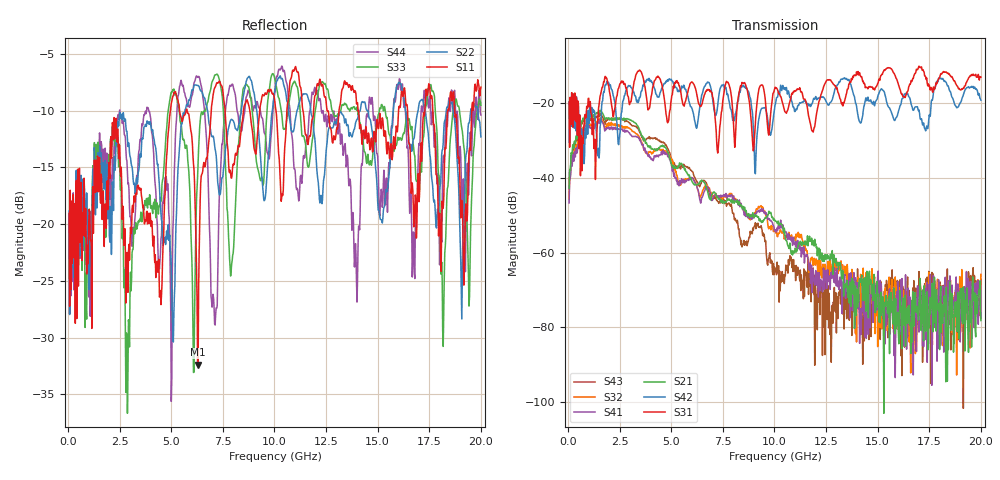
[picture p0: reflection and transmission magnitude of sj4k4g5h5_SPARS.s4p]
! FILE: E:\users\goganessyan\GBX_Backplane\FR408_backplane\1m_INBOUND_FEXT\sj4k4g5h5_SPARS.s4p
# MHZ S RI R 50.00
! FREQ  S11  S12  S13  S14
!  S21  S22  S23  S24
!  S31  S32  S33  S34
!  S41  S42  S43  S44
!  REAL  IMAG  REAL  IMAG  REAL  IMAG  REAL  IMAG
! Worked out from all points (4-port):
!   799 points, 50 MHz to 20 GHz, reference 50 ohm
!   strongest paths, dB at 50 MHz, 5.025 GHz, 10.03 GHz, 15.03 GHz, 20 GHz:
!     S31: -19.7, -18.0, -15.8, -14.5, -13.1
!     S42: -19.7, -14.0, -20.7, -17.8, -19.2
!     S21: -42.8, -36.8, -51.5, -71.4, -78.2
!     S41: -46.7, -37.2, -54.1, -65.0, -77.5
!     S32: -45.6, -35.0, -53.9, -71.4, -65.8
!     S43: -42.8, -35.3, -64.3, -68.4, -67.1
!   lowest |S11| = -32.4 dB at 6.275 GHz (marker M1), VSWR 1.05, Z = 51.9 - j1.58 ohm
!   |S11| at or under -10 dB: start of sweep to 4.959 GHz; 5.768 GHz to 6.936 GHz (1.168 GHz wide, 18.4 % of centre); 14.05 GHz to 16.01 GHz (1.965 GHz wide, 13.1 % of centre)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
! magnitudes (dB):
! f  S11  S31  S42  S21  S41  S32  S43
! 50 MHz  -19.0  -19.7  -19.7  -42.8  -46.7  -45.6  -42.8
! 1.55 GHz  -16.8  -18.2  -26.4  -21.9  -24.4  -23.9  -22.7
! 5.1 GHz  -8.7  -15.5  -14.8  -37.5  -38.7  -35.8  -36.5
! 6.275 GHz  -32.4  -18.7  -25.5  -41.7  -43.1  -43.1  -41.2
! 7.15 GHz  -7.8  -25.6  -23.4  -44.1  -44.6  -44.9  -45.3
! 12.75 GHz  -11.7  -14.2  -19.6  -61.6  -66.4  -65.2  -89.3
! 20 GHz  -7.9  -13.1  -19.2  -78.2  -77.5  -65.8  -67.1
